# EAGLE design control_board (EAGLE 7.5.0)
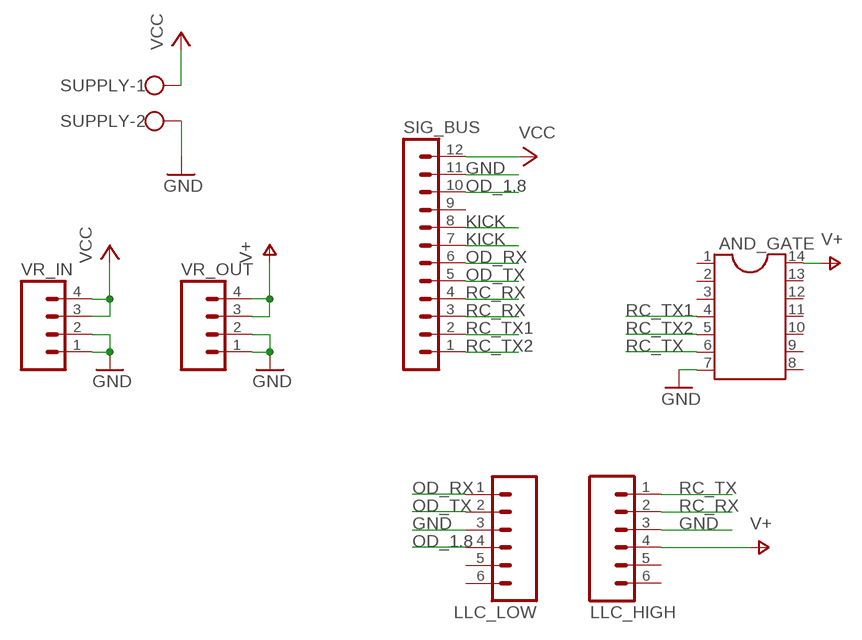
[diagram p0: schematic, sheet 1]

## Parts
AND_GATE  DIL14S  [SOCKET-14]
LLC_HIGH  M06  [06P]
LLC_LOW  M06  [06P]
SIG_BUS  MA12-1  [MA12-1]
SUPPLY  W237-102  [W237-102]
VR_IN  M04  [04P]
VR_OUT  M04  [04P]

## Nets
GND: AND_GATE.7 LLC_HIGH.3 LLC_LOW.3 SIG_BUS.11 SUPPLY.2 VR_IN.1 VR_IN.2 VR_OUT.1 VR_OUT.2
KICK: SIG_BUS.7 SIG_BUS.8
OD_1.8: LLC_LOW.4 SIG_BUS.10
OD_RX: LLC_LOW.1 SIG_BUS.6
OD_TX: LLC_LOW.2 SIG_BUS.5
RC_RX: LLC_HIGH.2 SIG_BUS.3 SIG_BUS.4
RC_TX: AND_GATE.6 LLC_HIGH.1
RC_TX1: AND_GATE.4 SIG_BUS.2
RC_TX2: AND_GATE.5 SIG_BUS.1
V+: AND_GATE.14 LLC_HIGH.4 VR_OUT.3 VR_OUT.4
VCC: SIG_BUS.12 SUPPLY.1 VR_IN.3 VR_IN.4
Unconnected: AND_GATE.1 AND_GATE.2 AND_GATE.3 AND_GATE.8 AND_GATE.9 AND_GATE.10 AND_GATE.11 AND_GATE.12 AND_GATE.13 LLC_HIGH.5 LLC_HIGH.6 LLC_LOW.5 LLC_LOW.6 SIG_BUS.9

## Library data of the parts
AND_GATE = ic-package:DIL14: Dual In Line / Socket
LLC_HIGH LLC_LOW = con-amp-quick:M06: AMP QUICK CONNECTOR; OC_FARNELL: unknown; OC_NEWARK: unknown
SIG_BUS = con-lstb:MA12-1: PIN HEADER; OC_FARNELL: unknown; OC_NEWARK: unknown
SUPPLY = con-wago-500:W237-102: WAGO SCREW CLAMP; MPN: 237-102; OC_FARNELL: unknown; OC_NEWARK: 70K9898
VR_IN VR_OUT = con-amp-quick:M04: AMP QUICK CONNECTOR; OC_FARNELL: unknown; OC_NEWARK: unknown

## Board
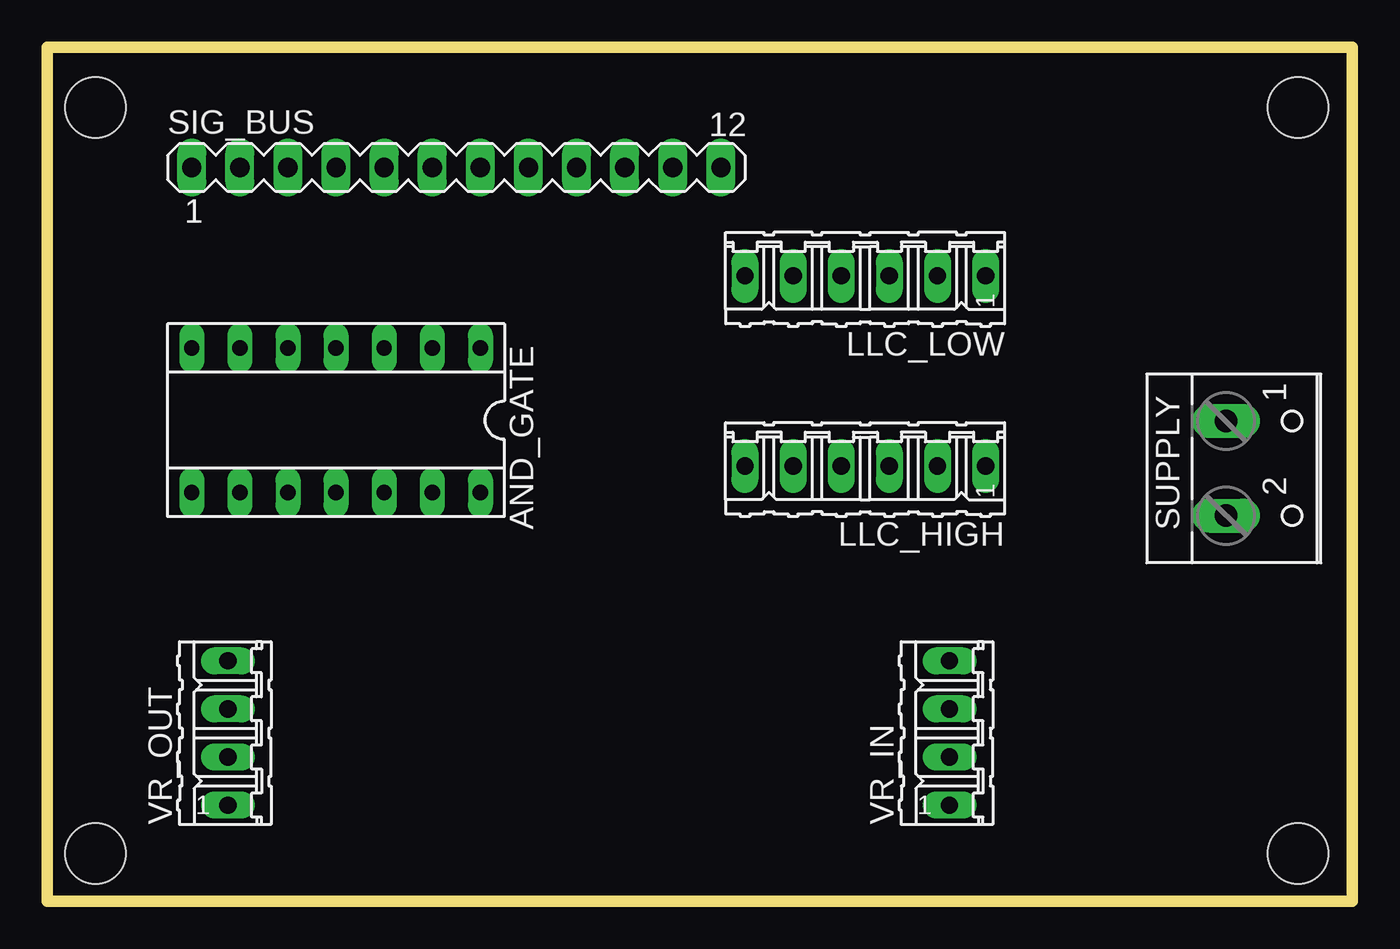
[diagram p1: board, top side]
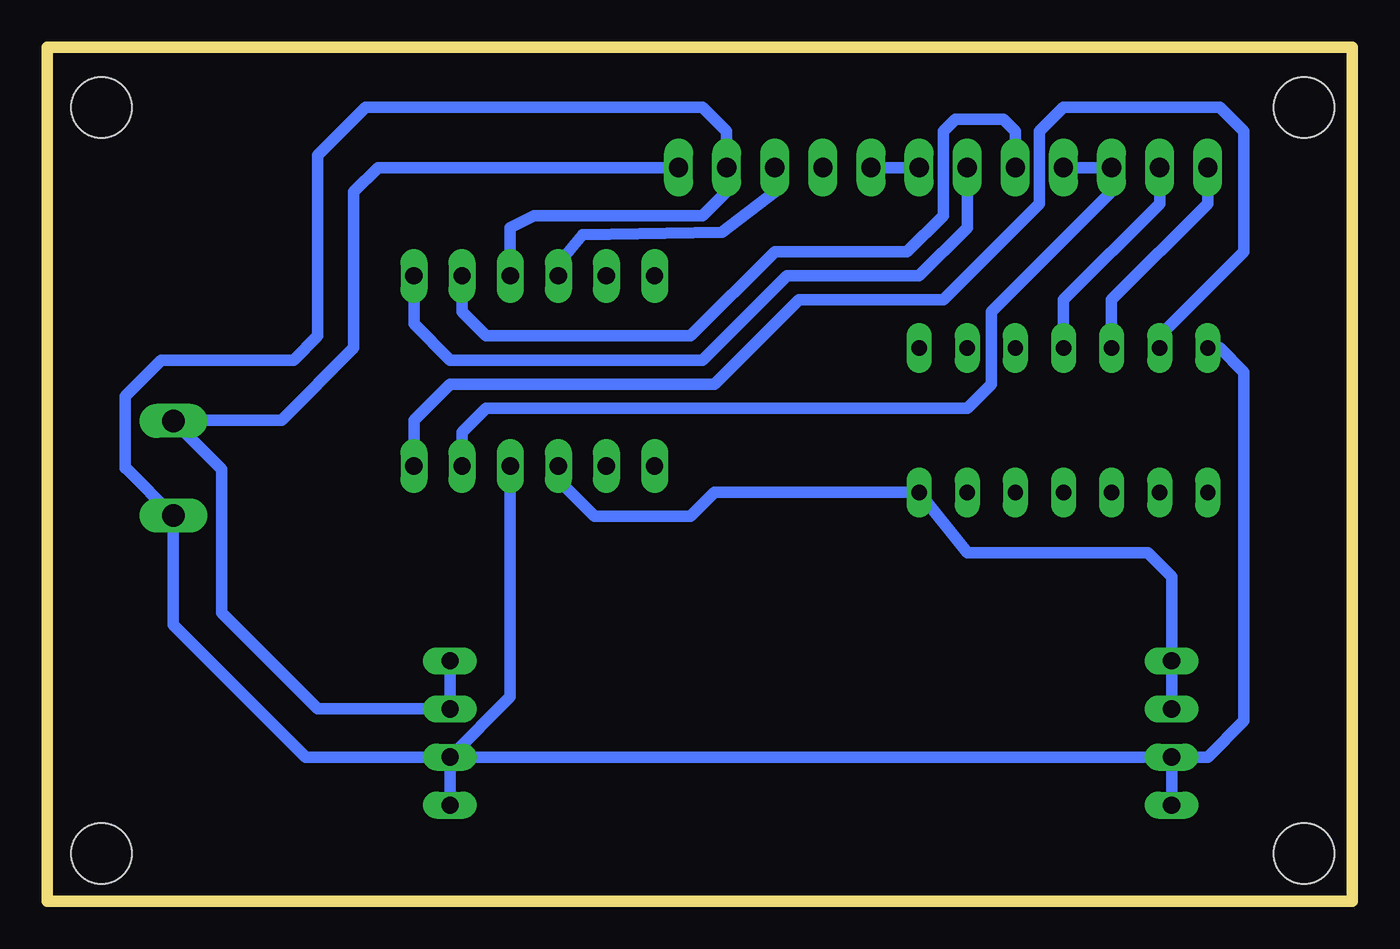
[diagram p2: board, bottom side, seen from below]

Size 68.89 x 45.08 mm. Coordinates in mm from the lower left corner, seen from the top.
Outline: 0,0 68.89,0 68.89,45.08 0,45.08 0,0
Copper layers (1*16): Top 0.035mm / dielectric 1.5mm / Bottom 0.035mm
Design rules "default *": minimum track width 24mil, minimum drill 16mil, track to track 8mil, track to pad 8mil, pad to pad 8mil, via to via 8mil, smd to smd 8mil, copper to edge 40mil, drill to drill 8mil, minimum pad ring 10mil, minimum via ring 8mil, stop-mask expansion 4mil, vias tented up to drill 0mil, thermal gap 10mil
Holes 3.2 mm at 2.54,2.54 66.04,2.54 66.04,41.91 2.54,41.91

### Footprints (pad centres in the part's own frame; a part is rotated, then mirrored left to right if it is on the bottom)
SOCKET-14 = drill 0.813 long: 1 -7.62,-3.81; 2 -5.08,-3.81; 3 -2.54,-3.81; 4 0,-3.81; 5 2.54,-3.81; 6 5.08,-3.81; 7 7.62,-3.81; 8 7.62,3.81; 9 5.08,3.81; 10 2.54,3.81; 11 0,3.81; 12 -2.54,3.81; 13 -5.08,3.81; 14 -7.62,3.81
06P = drill 0.914 long: 1 -6.35,0; 2 -3.81,0; 3 -1.27,0; 4 1.27,0; 5 3.81,0; 6 6.35,0
MA12-1 = drill 1.016 long: 1 -13.97,0; 2 -11.43,0; 3 -8.89,0; 4 -6.35,0; 5 -3.81,0; 6 -1.27,0; 7 1.27,0; 8 3.81,0; 9 6.35,0; 10 8.89,0; 11 11.43,0; 12 13.97,0
W237-102 = drill 1.194 long: 1 -2.5,-1.27; 2 2.5,-1.27
04P = drill 0.914 long: 1 -3.81,0; 2 -1.27,0; 3 1.27,0; 4 3.81,0

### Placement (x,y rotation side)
AND_GATE  15.24,25.4 180 top
LLC_HIGH  43.18,22.99 180 top
LLC_LOW  43.18,33.02 180 top
SIG_BUS  21.59,38.73 0 top
SUPPLY  63.5,22.86 270 top
VR_IN  47.62,8.89 90 top
VR_OUT  9.53,8.89 90 top

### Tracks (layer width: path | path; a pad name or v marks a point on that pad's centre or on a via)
GND
  Bottom 0.61: VR_IN.2 VR_IN.1 | VR_OUT.2 10,7.62 | 44.45,34.04 LLC_LOW.3 44.45,35.56 43.18,36.2 34.29,36.2 33.02,37.47 SIG_BUS.11 33.02,40.64 34.29,41.91 52.07,41.91 54.61,39.37 54.61,29.84 55.88,28.57 62.87,28.57 64.77,26.67 64.77,22.86 64.73,22.86 SUPPLY.2 | AND_GATE.7 6.99,29.21 5.71,27.94 5.71,9.53 7.62,7.62 VR_OUT.2 | VR_IN.2 VR_OUT.2 | LLC_HIGH.3 44.45,10.79 VR_IN.2 | SUPPLY.2 62.23,14.61 55.24,7.62 VR_IN.2 | 62.27,20.32 SUPPLY.2 | VR_OUT.1 VR_OUT.2
KICK
  Bottom 0.61: SIG_BUS.7 SIG_BUS.8
OD_1.8
  Bottom 0.61: LLC_LOW.4 41.91,33.66 40.64,35.18 33.27,35.31 30.48,37.47 SIG_BUS.10
OD_RX
  Bottom 0.61: SIG_BUS.6 20.32,35.56 22.86,33.02 29.84,33.02 34.29,28.57 47.62,28.57 49.53,30.48 LLC_LOW.1
OD_TX
  Bottom 0.61: SIG_BUS.5 17.78,40.64 18.41,41.27 20.95,41.27 21.59,40.64 21.59,36.2 23.5,34.29 30.48,34.29 34.92,29.84 45.72,29.84 46.99,31.11 LLC_LOW.2
RC_RX
  Bottom 0.61: SIG_BUS.4 SIG_BUS.3 12.7,37.47 19.05,31.11 19.05,27.3 20.32,26.04 45.72,26.04 46.99,24.77 LLC_HIGH.2
RC_TX
  Bottom 0.61: AND_GATE.6 10.16,29.84 5.71,34.29 5.71,40.64 6.99,41.91 15.24,41.91 16.51,40.64 16.51,36.83 21.59,31.75 29.21,31.75 33.66,27.3 47.62,27.3 49.53,25.4 LLC_HIGH.1
RC_TX1
  Bottom 0.61: SIG_BUS.2 10.16,36.83 15.24,31.75 AND_GATE.4
RC_TX2
  Bottom 0.61: SIG_BUS.1 7.62,36.83 12.7,31.75 AND_GATE.5
V+
  Bottom 0.61: VR_OUT.3 VR_OUT.4 9.53,17.14 10.79,18.41 20.32,18.41 AND_GATE.14 33.66,21.59 34.92,20.32 40.01,20.32 41.91,22.23 LLC_HIGH.4
VCC
  Bottom 0.61: SIG_BUS.12 51.44,38.73 52.7,37.47 52.7,29.21 56.52,25.4 62.19,25.4 SUPPLY.1 59.69,22.82 59.69,15.24 54.61,10.16 VR_IN.3 VR_IN.4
